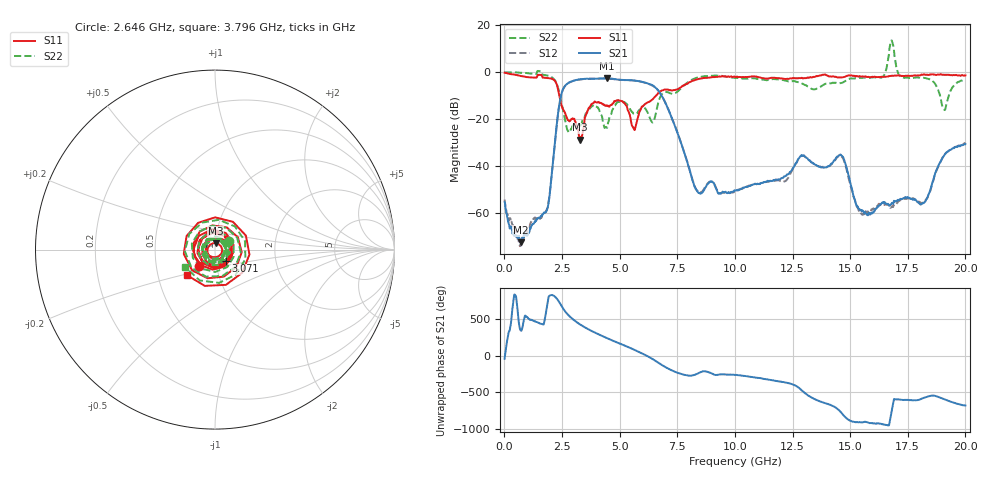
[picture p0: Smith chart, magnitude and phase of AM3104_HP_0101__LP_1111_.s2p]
!Created with skrf (http://scikit-rf.org).
# Hz S RI R 50.0
!freq ReS11 ImS11 ReS21 ImS21 ReS12 ImS12 ReS22 ImS22
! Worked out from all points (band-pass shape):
!   1601 points, 10 MHz to 20 GHz, reference 50 ohm
!   highest |S21| = -2.61 dB at 4.458 GHz (marker M1); lowest = -72.7 dB at 709.6 MHz (marker M2)
!   |S21| within 3 dB of the highest: 2.652 GHz to 6.428 GHz (3.775 GHz wide, 83.2 % of centre)
!   lowest |S11| = -28.8 dB at 3.283 GHz (marker M3), VSWR 1.08, Z = 50.3 + j3.64 ohm
!   |S11| at or under -10 dB: 2.382 GHz to 6.58 GHz (4.198 GHz wide, 93.7 % of centre)
!   |S22| runs from -25.8 to 13.6 dB; largest |S21 - S12| = 0.083
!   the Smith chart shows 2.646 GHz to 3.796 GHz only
!   S11 on the Smith chart (normalised r, x): 2.646 GHz: 0.82, -0.15; 3.071 GHz: 1.12, -0.15; 3.796 GHz: 0.70, -0.21
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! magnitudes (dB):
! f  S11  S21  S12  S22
! 10 MHz  -0.2  -55.5  -54.4  -0.1
! 709.6 MHz  -1.6  -72.7  -74.2  -0.2
! 1.859 GHz  -2.5  -58.4  -58.3  -1.4
! 2.371 GHz  -9.5  -14.5  -14.6  -8.3
! 2.646 GHz  -17.9  -5.7  -5.7  -20.9
! 3.071 GHz  -21.0  -3.4  -3.4  -22.8
! 3.283 GHz  -28.8  -3.0  -3.1  -22.9
! 3.346 GHz  -27.5  -2.9  -3.0  -22.1
! 3.796 GHz  -13.5  -2.8  -2.8  -14.3
! 4.458 GHz  -14.2  -2.6  -2.6  -23.8
! 4.958 GHz  -11.9  -3.2  -3.2  -12.5
! 5.62 GHz  -24.2  -3.5  -3.5  -17.7
! 6.682 GHz  -8.8  -7.8  -7.9  -12.8
! 8.368 GHz  -3.0  -50.9  -50.6  -2.2
! 10.01 GHz  -2.0  -50.6  -51.0  -2.4
! 13.34 GHz  -2.2  -38.6  -38.6  -7.1
! 14.62 GHz  -2.2  -35.5  -35.9  -4.6
! 15.45 GHz  -1.8  -59.0  -59.4  -2.4
! 16.68 GHz  -1.7  -56.7  -57.3  7.3
! 18.19 GHz  -1.0  -55.9  -55.9  -2.4
! 19.06 GHz  -1.0  -35.7  -35.6  -15.7
! 20 GHz  -1.3  -30.7  -30.3  -3.0
